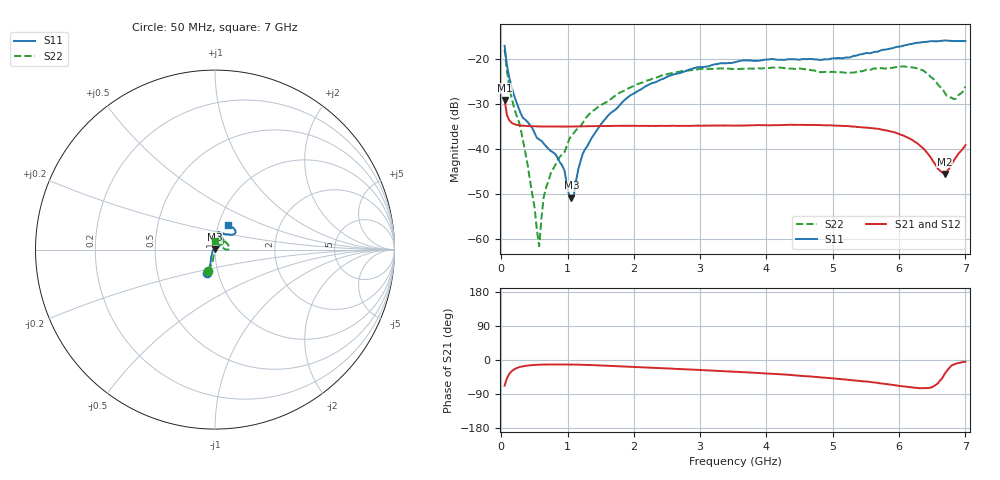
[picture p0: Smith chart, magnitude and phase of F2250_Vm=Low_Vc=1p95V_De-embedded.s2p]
! Integrated Device Technology
! Corporate Headquarters
! 6024 Silver Creek Valley Road
! San Jose, CA 95138  USA
! Phone:  1-408-284-8200
! Toll Free:  1-800-223-1366
! Webpage:  http://www.idt.com/
! Timing and RF Division
! 515 Groton Road, Suite 102
! Westford, MA 01886-6024
! Device:  F2250
! Description: Voltage Variable RF Attenuator
! Frequency:  50.0 -  6000.00 MHz
! Package:  3x3 mm Thin QFN Plastic Package: 16 pin
! Ports:  2 RF, 3 DC
!  Pin  1  = GND
!  Pin  2  = NC
!  Pin  3  = RF1  = Port 1
!  Pin  4  = NC
!  Pin  5  = GND
!  Pin  6  = GND
!  Pin  7  = GND
!  Pin  8  = GND
!  Pin  9  = NC
!  Pin 10  = RF2  = Port 2
!  Pin 11  = NC
!  Pin 12  = GND
!  Pin 13  = GND
!  Pin 14  = VCNTRL
!  Pin 15  = VDD
!  Pin 16  = VMODE
! Vcntrl:  1.950 Volts
! Vmode:  +0.000 Volts
! Vdd:  +3.30  Volts
! Current:  1.183 mA
! Data:  The device was measured on a the F2250 evaluation board which has
!  individual transmission lines to the RF pins.  Data was collected
!  using a calibrated network analyzer.  The evaluation board was
!  de-embedded using a TRL calibration technique.
!  The reference plane is the edge of the package pin.
! Misc:  SN 10
!  Action Tracker AT0258
! Date Measured:  2014-11-26
! Date:  2015-10-15  MJV
! Note:
!  Integrated Device Technology supplies this data as a sample of measured
!  data at the package pin for this product.  Your particular data for this
!  product may vary.
!  Data was taken at 25 degrees C.
!  Integrated Device Technology reserves the right to change this data at anytime.
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# GHz S dB R 50
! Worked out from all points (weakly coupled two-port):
!   201 points, 50 MHz to 7 GHz, reference 50 ohm
!   highest |S21| = -29.20 dB at 50 MHz (marker M1); lowest = -45.6 dB at 6.687 GHz (marker M2)
!   lowest |S11| = -50.9 dB at 1.058 GHz (marker M3), VSWR 1.01, Z = 49.9 + j0.242 ohm
!   |S11| at or under -10 dB: start of sweep to end of sweep
!   |S22| runs from -61.6 to -18.0 dB; largest |S21 - S12| = 6.1e-05
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0.05  -17.18 -108.6  -29.20 -67.5  -29.20 -67.5  -18.02 -107.2
0.1195  -24.20 -111.7  -33.71 -36.9  -33.71 -36.9  -26.17 -101.7
0.22375  -29.51 -122.0  -34.69 -21.9  -34.69 -22.0  -32.37 -102.7
0.29325  -32.20 -127.5  -34.87 -17.9  -34.87 -17.8  -35.60 -97.1
0.3975  -34.10 -141.4  -34.99 -14.7  -34.99 -14.7  -43.56 -93.2
0.50175  -36.52 -149.5  -35.04 -13.0  -35.05 -13.0  -53.07 -88.8
0.57125  -37.97 -160.3  -35.07 -12.4  -35.07 -12.4  -61.65 -21.0
0.64075  -38.89 -161.0  -35.09 -12.0  -35.09 -12.0  -50.70 33.5
0.6755  -39.47 -163.5  -35.09 -11.9  -35.09 -11.9  -48.68 36.5
0.91875  -43.76 158.3  -35.11 -11.8  -35.11 -11.8  -41.27 40.4
1.05775  -50.92 121.3  -35.10 -12.0  -35.10 -12.0  -37.09 43.9
1.0925  -50.56 88.6  -35.09 -12.1  -35.09 -12.1  -36.57 41.5
1.2315  -41.06 43.4  -35.04 -12.6  -35.05 -12.6  -34.22 33.0
1.6485  -32.09 41.8  -34.98 -15.3  -34.97 -15.4  -29.05 37.5
2.37825  -24.88 47.2  -34.95 -21.2  -34.95 -21.3  -24.02 42.3
3.525  -20.81 72.4  -34.90 -30.9  -34.90 -30.9  -22.35 66.7
4.7065  -20.17 72.3  -34.74 -44.2  -34.74 -44.2  -22.67 67.6
5.85325  -17.82 40.4  -36.12 -64.5  -36.12 -64.6  -22.08 14.9
6.33975  -16.40 40.9  -39.67 -74.4  -39.68 -74.4  -22.52 0.7
6.68725  -15.99 48.8  -45.61 -36.8  -45.59 -36.6  -27.59 21.0
6.82625  -16.14 53.5  -42.64 -11.8  -42.58 -11.7  -29.02 52.3
7  -16.12 63.2  -39.22 -4.6  -39.19 -4.7  -26.22 89.4
